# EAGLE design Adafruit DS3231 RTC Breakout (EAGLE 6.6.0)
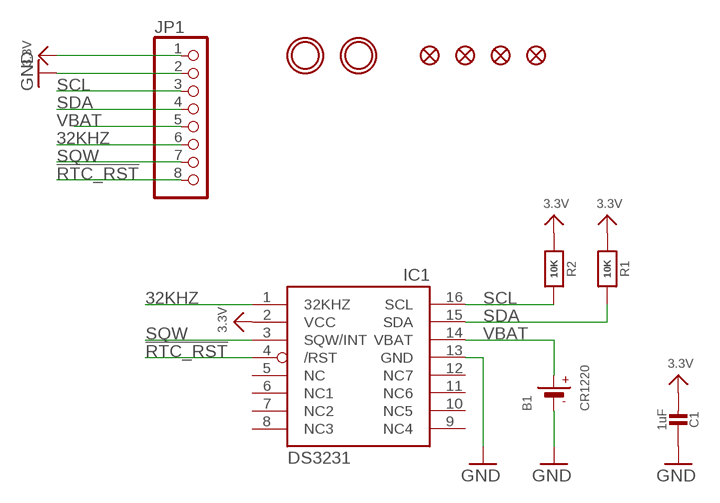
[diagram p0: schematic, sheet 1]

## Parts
B1  CR1220  BATTERYCR1220_SMT  [CR1220]
C1  1uF  CAP_CERAMIC0805-NOOUTLINE  [0805-NO]
FID1  FIDUCIAL""  [FIDUCIAL_1MM]
FID2  FIDUCIAL""  [FIDUCIAL_1MM]
FID3  FIDUCIAL""  [FIDUCIAL_1MM]
FID4  FIDUCIAL""  [FIDUCIAL_1MM]
IC1  DS3231/SO  [SO16W]
JP1  HEADER-1X870MIL  [1X08_ROUND_70]
R1  10K  RESISTOR0805_NOOUTLINE  [0805-NO]
R2  10K  RESISTOR0805_NOOUTLINE  [0805-NO]
U$6  MOUNTINGHOLE2.5  [MOUNTINGHOLE_2.5_PLATED]
U$7  MOUNTINGHOLE2.5  [MOUNTINGHOLE_2.5_PLATED]

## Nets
3.3V: C1.2 IC1.2(VCC) JP1.1 R1.1 R2.1
32KHZ: IC1.1(32KHZ) JP1.6
!RTC_RST: IC1.4(/RST) JP1.8
GND: B1.- C1.1 IC1.13(GND) JP1.2
SCL: IC1.16(SCL) JP1.3 R2.2
SDA: IC1.15(SDA) JP1.4 R1.2
SQW: IC1.3(SQW/INT) JP1.7
VBAT: B1.+$1(+) IC1.14(VBAT) JP1.5
Unconnected: IC1.5(NC) IC1.6(NC1) IC1.7(NC2) IC1.8(NC3) IC1.9(NC4) IC1.10(NC5) IC1.11(NC6) IC1.12(NC7)

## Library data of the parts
B1 = microbuilder:BATTERY: CR1220 SMT - Digikey: 3001K-ND
C1 = microbuilder:CAP_CERAMIC: Ceramic Capacitors
FID1-FID4 = microbuilder:FIDUCIAL: Fiducial Alignment Points; BOM: EXCLUDE
IC1 = adafruit:DS3231
JP1 = microbuilder:HEADER-1X8: PIN HEADER
R1 R2 = microbuilder:RESISTOR: Resistors
U$6 U$7 = microbuilder:MOUNTINGHOLE: Mounting Hole; BOM: EXCLUDE

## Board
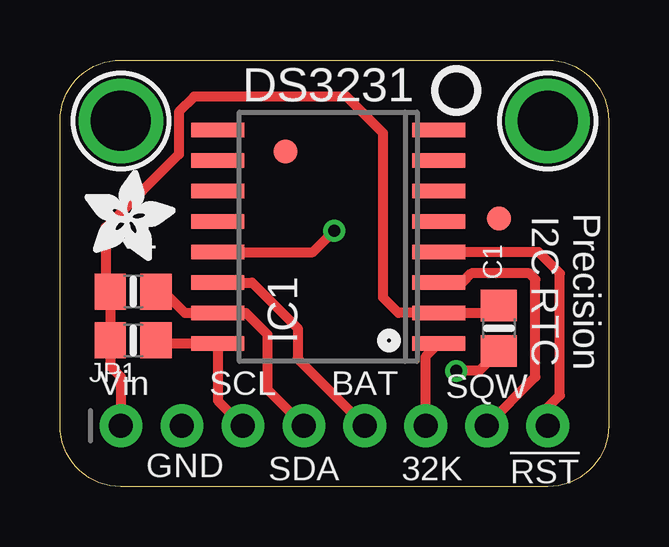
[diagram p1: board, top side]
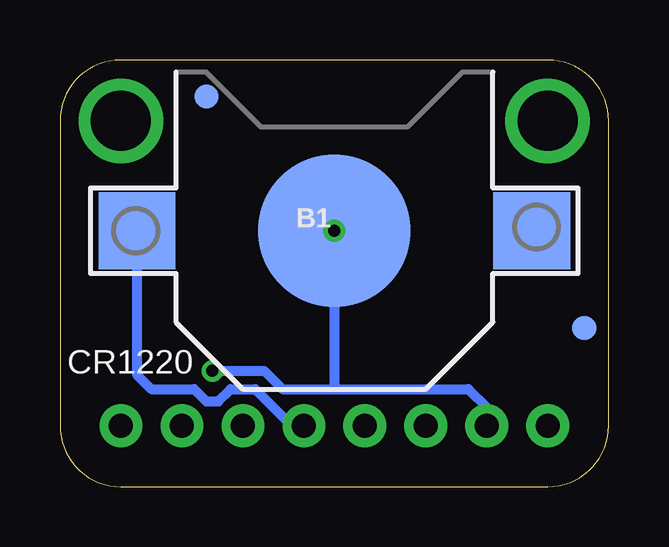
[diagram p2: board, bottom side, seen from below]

Size 22.86 x 17.78 mm. Coordinates in mm from the lower left corner, seen from the top.
Outline: 2.54,17.78 20.32,17.78 arc-90 22.86,15.24 22.86,2.54 arc-90 20.32,0 2.54,0 arc-90 0,2.54 0,15.24 arc-90 2.54,17.78
Copper layers (1*16): Top 0.035mm / dielectric 1.5mm / Bottom 0.035mm
Design rules "adafruit": minimum track width 8mil, minimum drill 15.5mil, track to track 8mil, track to pad 8mil, pad to pad 8mil, via to via 8mil, smd to smd 8mil, copper to edge 10mil, drill to drill 8mil, minimum pad ring 10mil, minimum via ring 8mil, stop-mask expansion 2mil, vias tented up to drill 20mil, thermal gap 10mil

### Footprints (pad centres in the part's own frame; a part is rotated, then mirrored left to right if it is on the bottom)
CR1220 = smd 3.2 x 3.2: +$1 -8.225,0; +$2 8.225,0 | smd 6.35 x 6.35: - 0,0
0805-NO = smd 1.3 x 1.5: 1 -0.95,0; 2 0.95,0
FIDUCIAL_1MM = smd 1 x 1: 1 0,0
SO16W = smd 0.6 x 2.2: 1 -4.445,-4.6; 2 -3.175,-4.6; 3 -1.905,-4.6; 4 -0.635,-4.6; 5 0.635,-4.6; 6 1.905,-4.6; 7 3.175,-4.6; 8 4.445,-4.6; 9 4.445,4.6; 10 3.175,4.6; 11 1.905,4.6; 12 0.635,4.6; 13 -0.635,4.6; 14 -1.905,4.6; 15 -3.175,4.6; 16 -4.445,4.6
1X08_ROUND_70 = drill 1 pad 1.778: 1 -8.89,0; 2 -6.35,0; 3 -3.81,0; 4 -1.27,0; 5 1.27,0; 6 3.81,0; 7 6.35,0; 8 8.89,0
MOUNTINGHOLE_2.5_PLATED = drill 2.5 pad 3.2: P$1 0,0

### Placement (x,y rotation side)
B1  11.43,10.67 0 bottom
C1  18.29,6.6 90 top
FID1  9.4,13.97 0 top
FID2  1.02,6.6 0 bottom
FID3  18.29,11.18 0 top
FID4  16.76,16.26 0 bottom
IC1  11.18,10.41 90 top
JP1  11.43,2.54 0 top
R1  3.05,8.13 0 top
R2  3.05,6.1 0 top
U$6  20.32,15.24 0 top
U$7  2.54,15.24 0 top
U$8  [ADAFRUIT_3.5MM]  1.02,9.4 0 top
U$9  [PCBFEAT-REV-040]  16.51,16.51 0 top

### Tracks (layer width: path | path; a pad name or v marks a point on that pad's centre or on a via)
3.3V
  Top 0.406: C1.2 18.09,7.24 IC1.2 14.1,7.24 13.46,7.87 13.46,14.73 11.94,16.26 5.59,16.26 4.95,15.62 4.95,13.84 1.91,10.79 1.91,8.32 R1.1 R2.1 2.1,5.01 2.54,4.57 JP1.1
32KHZ
  Top 0.406: JP1.6 15.24,5.43 IC1.1
!RTC_RST
  Top 0.406: JP1.8 20.32,3.3 20.83,3.81 20.83,8.89 19.94,9.78 IC1.4
GND  (via drill 0.5)
  Top 0.406: IC1.13 10.54,9.78 B1.- | C1.1 17.46,4.83 v16.51,4.83
  Bottom 0.406: 11.94,8.89 11.94,10.67 B1.- 11.43,4.06 | JP1.2 5.08,3.3 5.84,4.06 11.43,4.06 | v16.51,4.83 14.35,4.83 13.59,4.06 11.43,4.06
  other vias: 11.43,10.67
SCL
  Top 0.406: JP1.3 6.58,3.58 IC1.16 4.12,5.97 R2.2
SDA
  Top 0.406: JP1.4 8.64,4.06 8.64,6.35 7.75,7.24 IC1.15 5.21,7.24 4.32,8.13 R1.2
SQW
  Top 0.406: JP1.7 19.81,4.57 19.81,8.64 19.56,8.89 17.14,8.89 16.76,8.51 IC1.3
VBAT
  Top 0.406: IC1.14 8,8.51 9.91,6.6 9.91,5.33 JP1.5
  Bottom 0.406: B1.+$1 19.66,4.67 19.05,4.06 17.27,4.06 16.76,3.56 16.26,3.56 15.75,4.06 14.73,4.06 13.21,2.54 JP1.5

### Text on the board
tPlace: DS3231 | Precision / I2C RTC | Vin | SCL | BAT | SQW | GND | SDA | 32K | !RST
bPlace: CR1220

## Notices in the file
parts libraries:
microbuilder: This work is placed in the public domain, and may be freely used for commercial and non-commercial work with the following conditions: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
